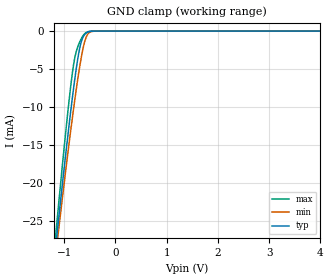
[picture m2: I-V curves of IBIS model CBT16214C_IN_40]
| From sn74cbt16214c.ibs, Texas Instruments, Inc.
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[Model]   CBT16214C_IN_40
Model_type  Input
Vinl=0.8
Vinh=2.0
| variable   typ   min   max
C_comp   2.18pF   1.55pF   2.90pF
[Temperature Range]   40   100   -40
| Ambient temperature   25   85   -40
[Voltage range]   4   4   4
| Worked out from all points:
|   GND clamp passes 1 mA (typ) near -0.64 V on its own axis
[GND Clamp]
| CBT16214C_IN_40
|   Voltage   I(typ)   I(min)   I(max)
-4V       -228.7mA   -212.7mA   -248.5mA
-1.17V    -28.73mA   -29.82mA   -27.27mA
-1.135V   -26.5mA    -27.79mA   -24.77mA
-1.105V   -24.61mA   -26.05mA   -22.65mA
-920mV    -13.36mA   -15.71mA   -10.21mA
-815mV    -7.535mA   -10.23mA   -4.436mA
-765mV    -5.059mA   -7.789mA   -2.763mA
-680mV    -1.806mA   -4.061mA   -1.212mA
-615mV    -615.5uA   -1.842mA   -473.8uA
-555mV    -205uA     -602.5uA   -131.9uA
-410mV    -6.4uA     -14.18uA   -1.367uA
4V        94.31pA    243.3pA    55.56pA
